(* Logix 5000 AddOnInstructionDefinition export AKD_Response_Assembly; software revision 20.04 *)

TYPE AKD_Status :   // All connections to the drive ethernet module are established and data is successfully transferring.
STRUCT
   Profile_In_Progress : BOOL;   // Profile Move In Progress
   Block_In_Execution : BOOL;   // Block In Execution
   On_Target_Position : BOOL;   // On Target Position (1=Current Position Equals Last Target Position)
   General_Fault : BOOL;   // General Fault
   Current_Direction : BOOL;   // Current Motor Direction (0=Reverse, 1=Forward)
   Home_Level : BOOL;   // Level of Home Input
   Reg_Level : BOOL;   // Level of Registration Input
   Enable : BOOL;   // State of Enable Output
   Fault_Input_Fault : BOOL;   // Fault Input Active
   Fwd_Limit : BOOL;   // Forward Input Active
   Rev_Limit : BOOL;   // Reverse Input Active
   Positive_Limit : BOOL;   // Positive Software Limit Exceeded
   Negative_Limit : BOOL;   // Negative Software Limit Exceeded
   FE_Fault : BOOL;   // Following Error Fault
   Block_Fault : BOOL;   // Block Execution Fault
   Load_Complete : BOOL;   // Command Message Successfully Loaded
END_STRUCT
END_TYPE

TYPE AKD_Control :   // Send Explicit Message
STRUCT
   Load_Data_Start_Profile : BOOL;   // Load Command Data / Start Profile Move
   Start_Block : BOOL;   // Execute Command block or block chain
   Incremental : BOOL;   // Incremental Position (0=Absolute, 1=Incremental)
   Direction : BOOL;   // Direction in Velocity Mode (0=Reverse, 1=Forward)
   Smooth_Stop : BOOL;   // Smooth / Controlled Stop w/ Deceleration
   Hard_Stop : BOOL;   // Hard / Immediate Stop
   Reg_Arm : BOOL;   // Arm the Registration Input
   Enable : BOOL;   // Enable Output
END_STRUCT
END_TYPE

TYPE AKD_Axis :   // Axis Data:
STRUCT
   Control : AKD_Control;   // Control bits to send to the drive
   Status : AKD_Status;   // Status bits received from the drive
   Input : AB:ETHERNET_MODULE_SINT_64Bytes:I:0;   // Data from the drive
   Output : AB:ETHERNET_MODULE_SINT_64Bytes:O:0;   // Data to the drive
   ResponseMsgType : SINT;   // Response type contained in latest IO response from drive. Used to check for errors
   CommandTimeout : INT;   // Time to allow for command response from drive. Dependent on scan rate and communicaiton rate
   PositionFeedback : DINT;   // Actual Position Value
   VelocityFeedback : DINT;   // Actual Velocity Value
END_STRUCT
END_TYPE

ADD_ON_INSTRUCTION AKD_Response_Assembly   (* revision 2.0 *)
VAR_IN_OUT
   Axis : AKD_Axis; {required}
END_VAR
VAR_OUTPUT
   Status_Word_1 : SINT; {access Read Only, visible}
   Executing_Block_Number : SINT; {access Read Only, visible}
   Status_Word_2 : SINT; {access Read Only, visible}
   Response_Type : SINT; {access Read Only, visible}
   Data : DINT; {access Read Only, visible}
   Actual_Position : DINT; {access Read Only, visible}
   Actual_Velocity : DINT; {access Read Only, visible}
   Motion_Status : DINT; {access Read Only, visible}
   Parameter_Attribute_Data : DINT; {access Read Only, visible}
   Attribute_To_Get : SINT; {access Read Only, visible}
   Map_Type : SINT; {access Read Only, visible}
   Ethernet_Command_Response_Error_Occurred : BOOL; {visible}
   Error_Code : SINT; {visible}
   Additional_Code : SINT; {visible}
END_VAR
VAR_INPUT
   Clear_Error_Status : BOOL; {visible}
END_VAR
VAR
   error_os : BOOL;
   clear_error_os : BOOL;
END_VAR

ROUTINE Logic   (* ladder *)
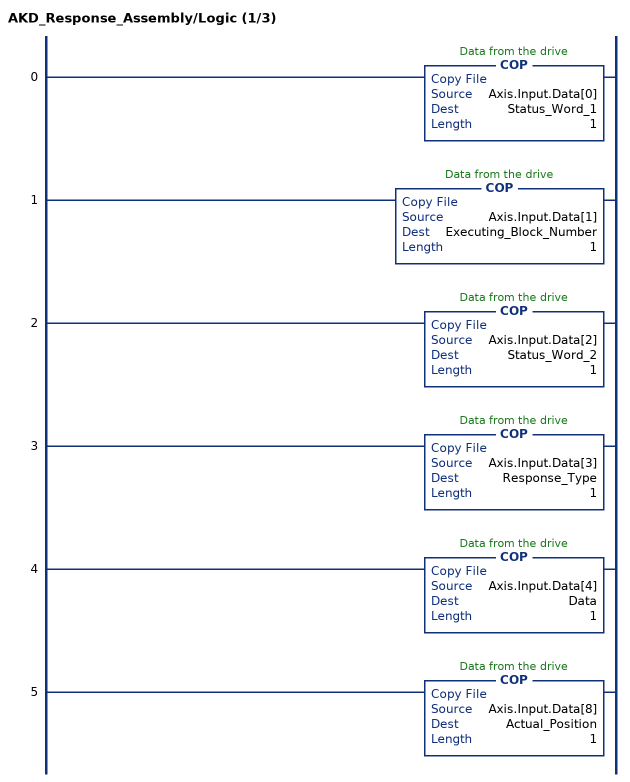
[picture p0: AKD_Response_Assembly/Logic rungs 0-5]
   0: COP(Axis.Input.Data[0],Status_Word_1,1);
   1: COP(Axis.Input.Data[1],Executing_Block_Number,1);
   2: COP(Axis.Input.Data[2],Status_Word_2,1);
   3: COP(Axis.Input.Data[3],Response_Type,1);
   4: COP(Axis.Input.Data[4],Data,1);
   5: COP(Axis.Input.Data[8],Actual_Position,1);
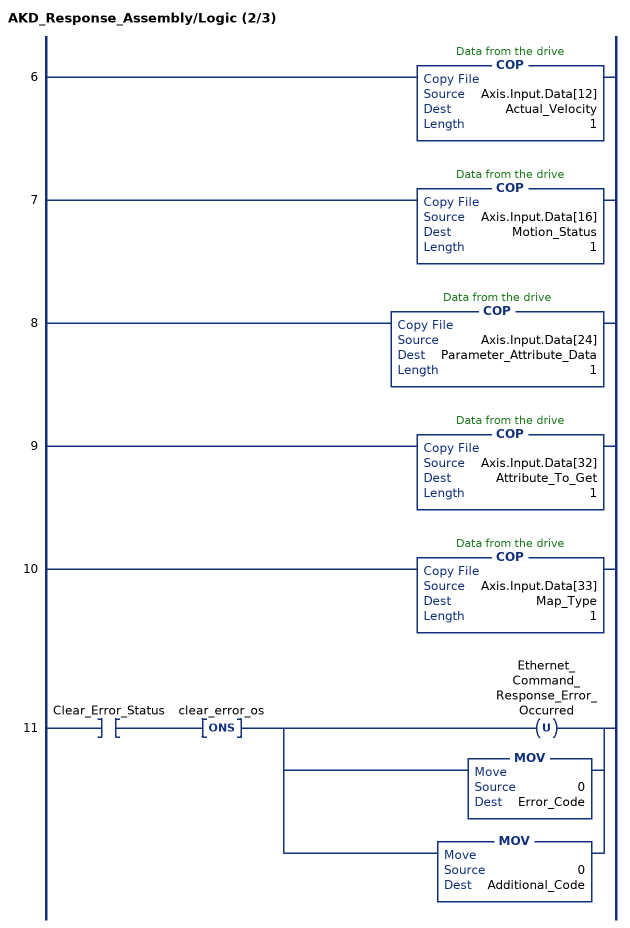
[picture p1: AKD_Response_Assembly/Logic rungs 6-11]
   6: COP(Axis.Input.Data[12],Actual_Velocity,1);
   7: COP(Axis.Input.Data[16],Motion_Status,1);
   8: COP(Axis.Input.Data[24],Parameter_Attribute_Data,1);
   9: COP(Axis.Input.Data[32],Attribute_To_Get,1);
   10: COP(Axis.Input.Data[33],Map_Type,1);
   11: XIC(Clear_Error_Status)ONS(clear_error_os)[OTU(Ethernet_Command_Response_Error_Occurred) ,[MOV(0,Error_Code) ,MOV(0,Additional_Code) ] ];
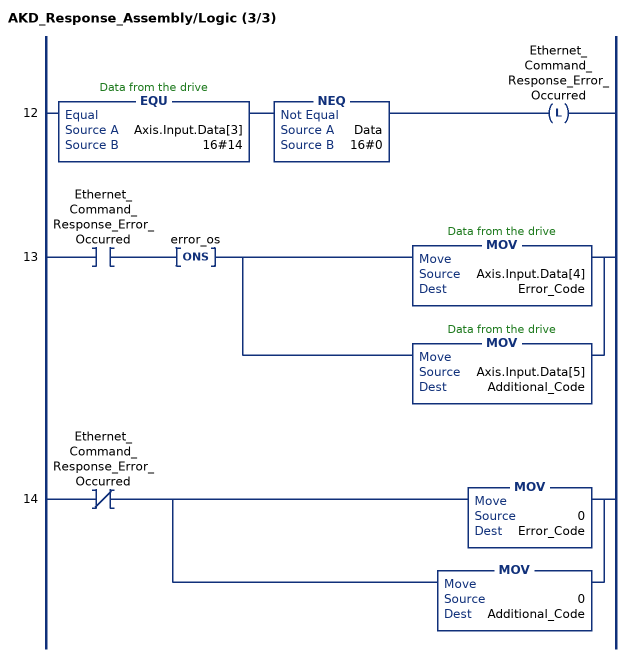
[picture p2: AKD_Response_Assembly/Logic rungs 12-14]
   12: EQU(Axis.Input.Data[3],16#14)NEQ(Data,16#0)OTL(Ethernet_Command_Response_Error_Occurred);
   13: XIC(Ethernet_Command_Response_Error_Occurred)ONS(error_os)[MOV(Axis.Input.Data[4],Error_Code) ,MOV(Axis.Input.Data[5],Additional_Code) ];
   14: XIO(Ethernet_Command_Response_Error_Occurred)[MOV(0,Error_Code) ,MOV(0,Additional_Code) ];
END_ROUTINE
END_ADD_ON_INSTRUCTION
